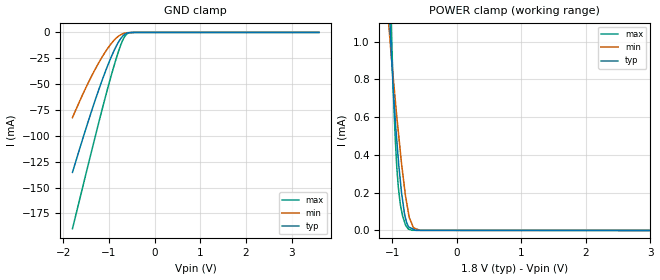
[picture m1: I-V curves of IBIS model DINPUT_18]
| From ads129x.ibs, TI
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|NOTES   Model TERM split into three Models TERM_18, TERM_2, and TERM_33
|   to accomodate voltage range of 1.65 V - 3.6V
|   TERM_18 operates in voltage range of 1.65 - 1.8 - 1.96
|   (specifically for ADS1294, ADS1296, and ADS1298 products)
|   TERM_2 operates in voltage range of 1.8 - 2.0 - 2.2
|   (specifically for ADS1291,ADS1292, ADS1292R, and ADS1299 products)
|   TERM_33 operates in voltage range of 3 - 3.3 - 3.6
|   (for all products)
|   DINPUT 1.8V Model
[Model]   DINPUT_18
Model_type   Input
|for ADS1291, ADS1292, ADS1294, ADS1296, and ADS1298 products
|Signals   DIN, CLKSEL, START, _CS, _RESET, _PWDN, RESV1
Vinl = 0.36
Vinh = 1.44
|   typ   min   max
|   (nom PVT)   (Fast PVT)   (slow PVT)
|C_comp from frequency sweep method (F=64MHz)
|C_comp   2.5452470e-12   1.8682050e-12   3.0942680e-12
|C_comp from LC tank measurement(L=1nH)
C_comp   1.762E-12   1.432E-12   2.090E-12
| Where   nom PVT is  Nominal Process, 1.8V, 27C
|   Fast PVT is Strong Process, 2V, -40C
|   Slow PVT is Weak Process, 1.65V, 85C
[Voltage Range]   1.8   1.65   2
[Temperature Range]   27   85   -40
[Power Clamp Reference]   1.8   1.65   2
[GND Clamp Reference]   0   0   0
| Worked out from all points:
|   GND clamp passes 1 mA (typ) near -0.62 V on its own axis
|   POWER clamp passes 1 mA (typ) near -1.02 V on its own axis
[GND Clamp]
|   Voltage   I(typ)   I(min)   I(max)
-1.8V     -135.3mA   -82.39mA   -189.7mA
-1.616V   -108.7mA   -63.88mA   -156.7mA
-1.379V   -75.57mA   -41.98mA   -114.3mA
-1.23V    -56.14mA   -29.74mA   -88.13mA
-1.062V   -35.84mA   -17.66mA   -59.61mA
-932.5mV  -21.81mA   -9.837mA   -38.75mA
-792.7mV  -9.398mA   -3.624mA   -18.42mA
-709mV    -4.1mA     -1.551mA   -8.389mA
-674.7mV  -2.584mA   -992.8uA   -5.261mA
-611mV    -858.6uA   -415.2uA   -1.62mA
-440mV    -12.33uA   -13.16uA   -11.39uA
3.595V    0A         0A         0A
[POWER Clamp]
|   Voltage   I(typ)   I(min)   I(max)
-1.8V     10.43mA    8.127mA    13.16mA
-1.051V   1.214mA    1.076mA    1.506mA
-1.037V   1.102mA    1.014mA    1.323mA
-1.017V   953.2uA    928.3uA    1.088mA
-954.5mV  588uA      692.9uA    491.3uA
-907.1mV  378.3uA    524.9uA    231.9uA
-870.3mV  246.8uA    400.7uA    128.7uA
-813.8mV  94.97uA    234.6uA    48.61uA
-753.5mV  23.33uA    100.5uA    8.199uA
-670.2mV  5.85uA     13.5uA     989.7nA
-565.3mV  691.6nA    574.1nA    965.3nA
3.595V    0A         0A         0A
